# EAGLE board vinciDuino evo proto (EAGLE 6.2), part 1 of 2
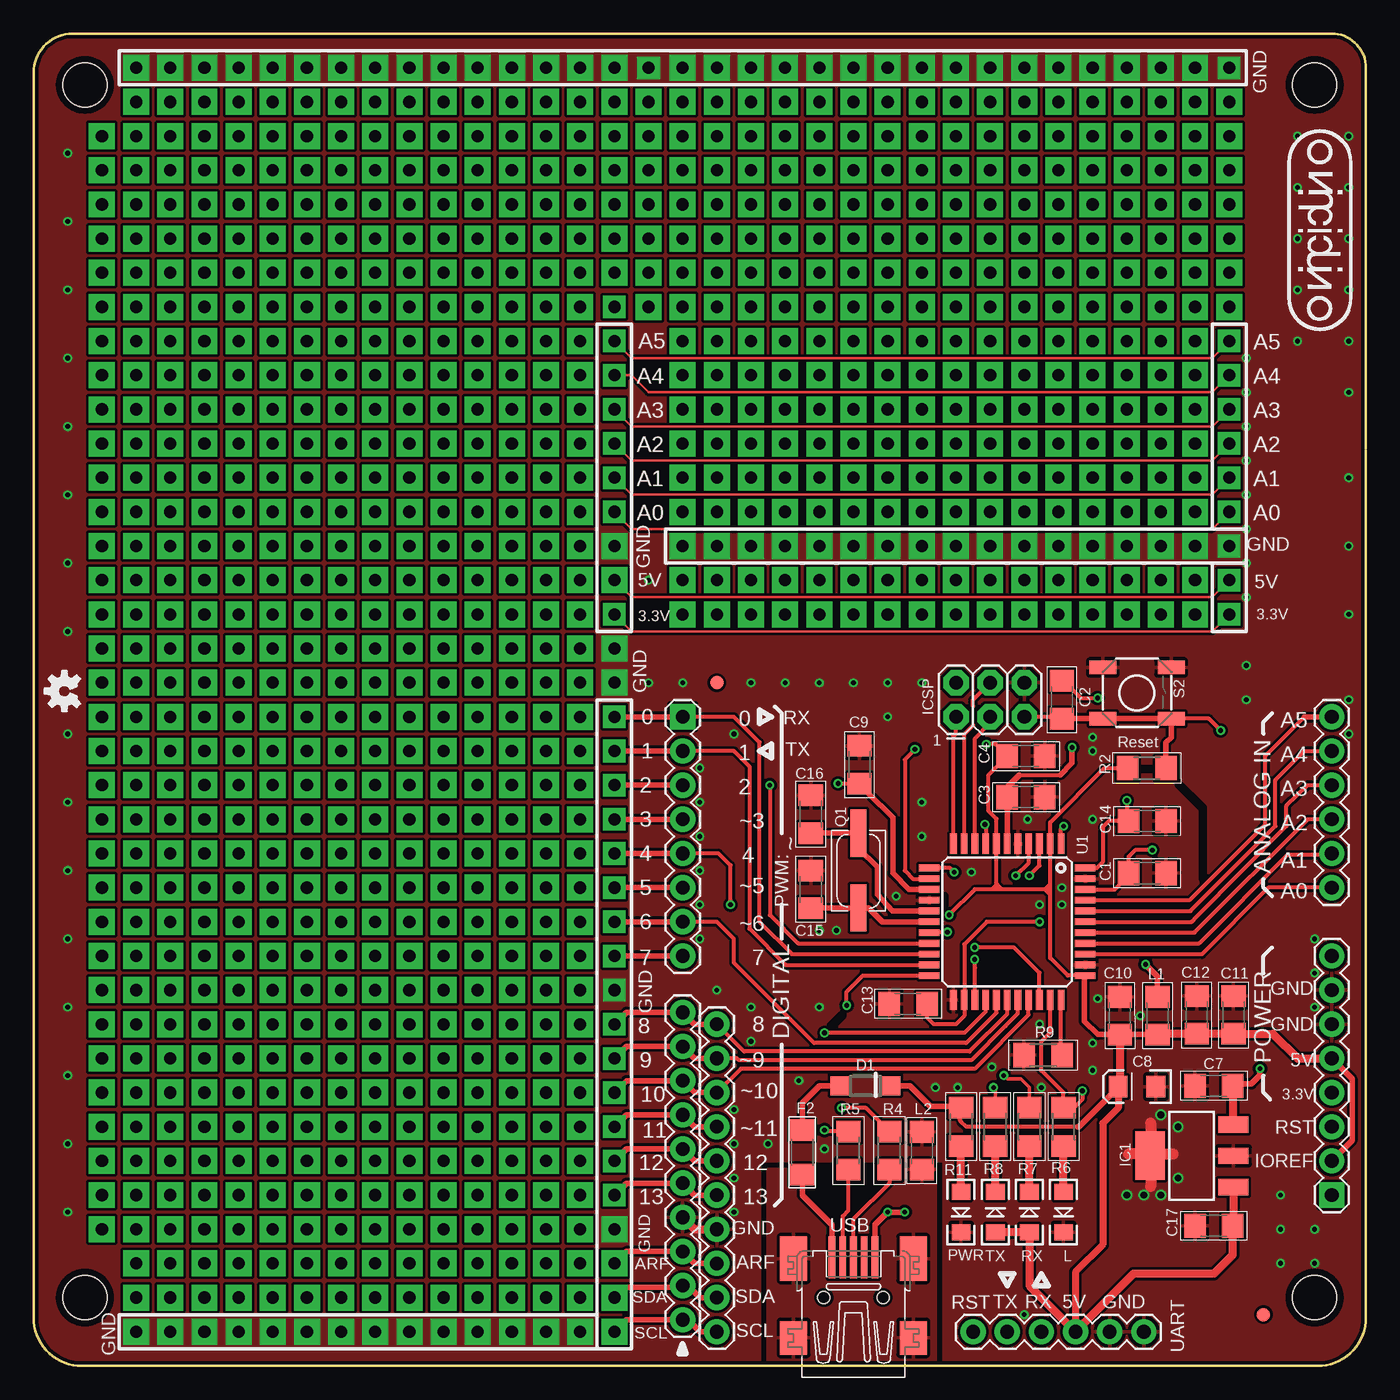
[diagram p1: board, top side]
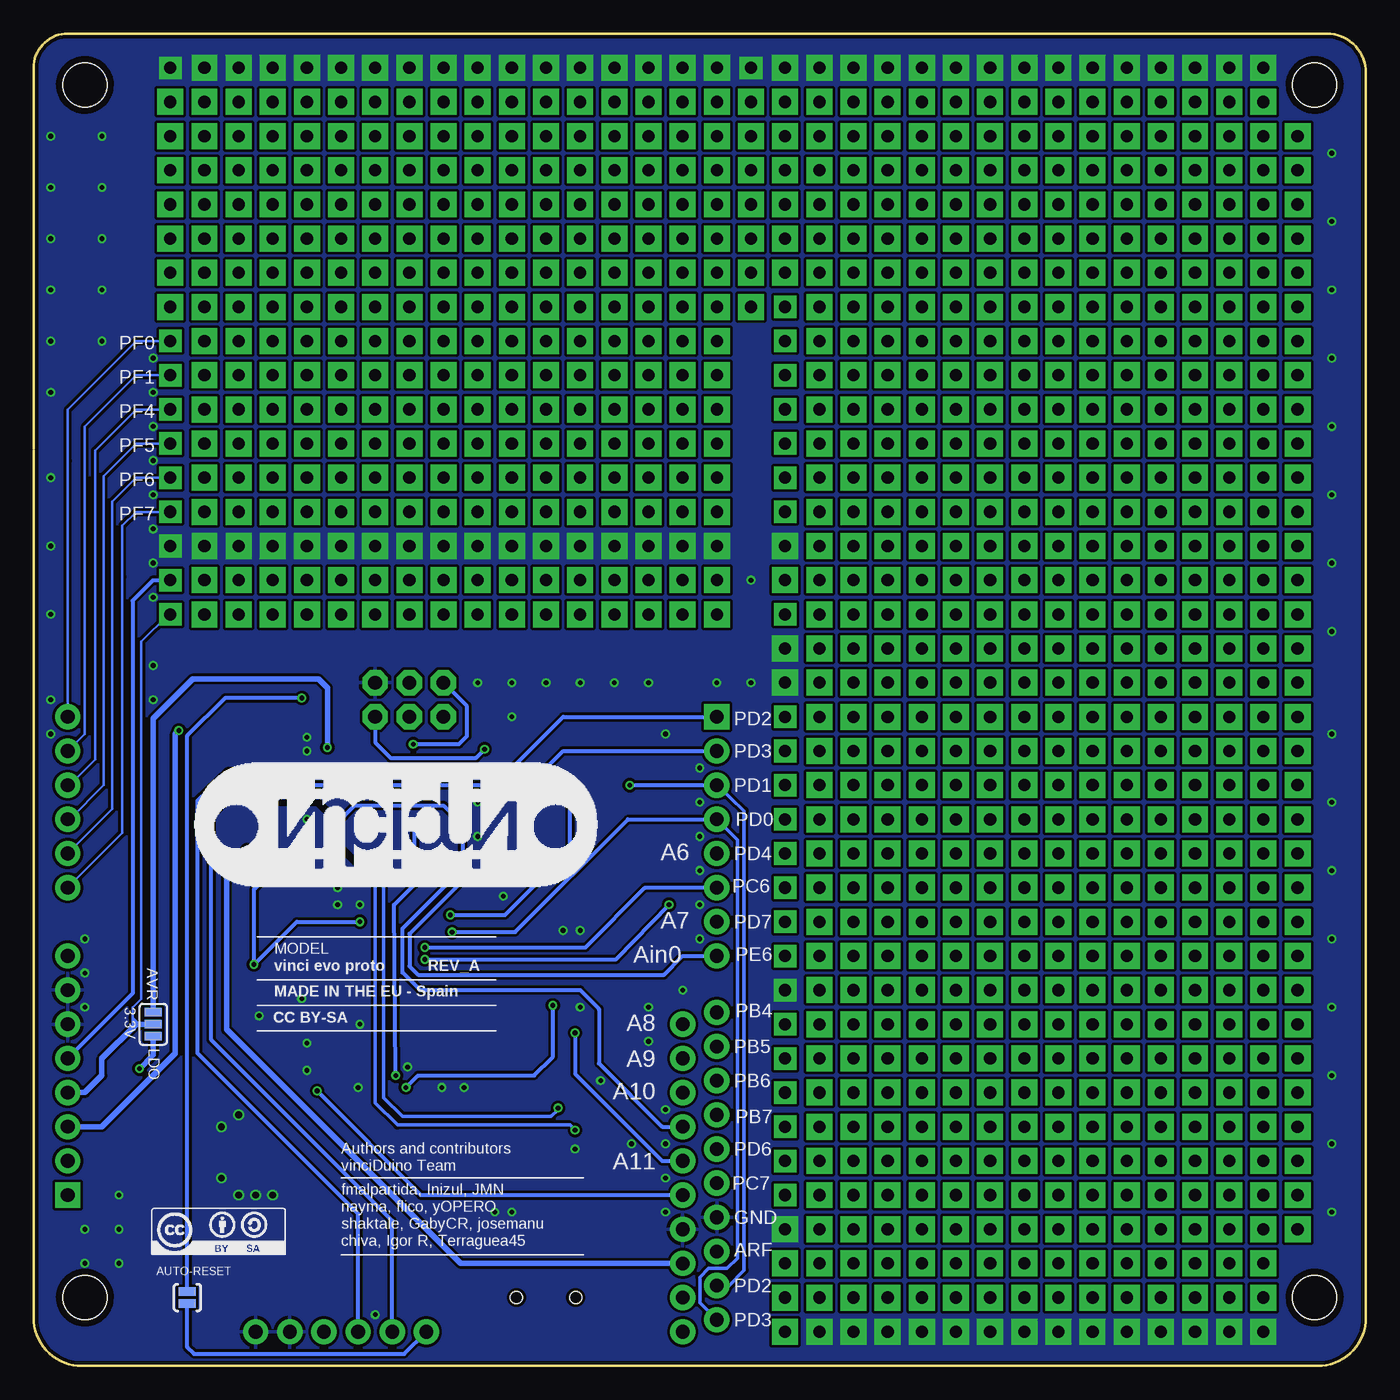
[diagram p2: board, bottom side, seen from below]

Size 99.06 x 99.06 mm. Coordinates in mm from the lower left corner, seen from the top.
Outline: 99.06,68.05 99.06,3.59 arc-90 95.47,0 3.59,0 arc-90 0,3.59 0,96.16 arc-90 2.9,99.06 96.52,99.06 arc-90 99.06,96.52 99.06,68.2
Copper layers (1*16): Top 0.0356mm / dielectric 1.5011mm / Bottom 0.0356mm
Design rules: minimum track width 6mil, minimum drill 0.35mm, track to track 8mil, track to pad 8mil, pad to pad 8mil, via to via 8mil, smd to smd 8mil, copper to edge 10mil, drill to drill 6mil, minimum pad ring 12mil, minimum via ring 6mil, stop-mask expansion 4mil, vias tented up to drill 25mil, thermal gap 10mil
Net classes: 1 vcc: width 0.254 mm; 2 usb: width 0.203 mm, clearance 0.508 mm
tRestrict: area 67.6,34.3 to 67.7,34.9; area 59.2,25.1 to 60.2,26.2; area 85.1,36.2 to 87,43.4; area 82.3,44.3 to 83.2,44.5
bRestrict: area 74.5,36.8 to 76.6,39.5; area 76.7,40.6 to 80.8,42

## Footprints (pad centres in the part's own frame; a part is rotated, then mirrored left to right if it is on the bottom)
SJ_3 = smd 0.635 x 1.27: 1 -0.889,0; 2 0,0; 3 0.889,0
SJ_2S-NO = smd 0.635 x 1.27: 1 -0.45,0; 2 0.45,0
1206 = smd 1.6 x 1.8: 1 -1.4,0; 2 1.4,0
EIA3216 = smd 1.4 x 1.6: A 1.4,0; C -1.4,0
SOD123 = smd 1.4 x 1.4: A 1.9,0; C -1.9,0
1206_PTC = smd 1.6 x 1.8: 1 -1.654,0; 2 1.654,0
SOT223 = smd 1.219 x 2.235: 1 -2.311,-3.099; 2 0,-3.099; 3 2.311,-3.099 | smd 3.6 x 2.2: 4 0,3.099
1X08@1 = drill 1.016 pad 1.88 square: 1 0,0 | drill 1.016 pad 1.88: 2 2.54,0; 3 5.08,0; 4 7.62,0; 5 10.16,0; 6 12.7,0; 7 15.24,0; 8 17.78,0
1X06@1 = drill 1.016 pad 1.88: 1 -6.35,0; 2 -3.81,0; 3 -1.27,0; 4 1.27,0; 5 3.81,0; 6 6.35,0
1X10 = drill 1.016 pad 1.88: 1 0,0; 2 2.54,0; 3 5.08,0; 4 7.62,0; 5 10.16,0; 6 12.7,0; 7 15.24,0; 8 17.78,0; 9 20.32,0; 10 22.86,0
2X3@1 = drill 1.016 pad 1.88 octagon: 1 0,0; 2 0,2.54; 3 2.54,0; 4 2.54,2.54; 5 5.08,0; 6 5.08,2.54
1X08 = drill 1.016 pad 1.88 square: 1 0,0 | drill 1.016 pad 1.88: 2 2.54,0; 3 5.08,0; 4 7.62,0; 5 10.16,0; 6 12.7,0; 7 15.24,0; 8 17.78,0
LED-1206 = smd 1.2 x 1.4: A -1.5,0; C 1.5,0
1206W = smd 1.6 x 1.8: 1 -1.4,0; 2 1.4,0
CSM-3X = smd 3.5 x 1.2: 1 2.775,0; 2 -2.775,0
R1206 = smd 1.6 x 1.803: 1 -1.422,0; 2 1.422,0
TACTILE_SWITCH_SMD@1 = smd 2 x 1: 1 -2.54,1.905; 2 2.54,1.905; 3 -2.54,-1.905; 4 2.54,-1.905
TQFP44 = smd 1.5 x 0.5: 1 -5.8,4; 2 -5.8,3.2; 3 -5.8,2.4; 4 -5.8,1.6; 5 -5.8,0.8; 6 -5.8,0; 7 -5.8,-0.8; 8 -5.8,-1.6; 9 -5.8,-2.4; 10 -5.8,-3.2; 11 -5.8,-4; 23 5.8,-4; 24 5.8,-3.2; 25 5.8,-2.4; 26 5.8,-1.6; 27 5.8,-0.8; 28 5.8,0; 29 5.8,0.8; 30 5.8,1.6; 31 5.8,2.4; 32 5.8,3.2; 33 5.8,4 | smd 0.5 x 1.5: 12 -4,-5.8; 13 -3.2,-5.8; 14 -2.4,-5.8; 15 -1.6,-5.8; 16 -0.8,-5.8; 17 0,-5.8; 18 0.8,-5.8; 19 1.6,-5.8; 20 2.4,-5.8; 21 3.2,-5.8; 22 4,-5.8; 34 4,5.8; 35 3.2,5.8; 36 2.4,5.8; 37 1.6,5.8; 38 0.8,5.8; 39 0,5.8; 40 -0.8,5.8; 41 -1.6,5.8; 42 -2.4,5.8; 43 -3.2,5.8; 44 -4,5.8
FIDUCIAL-1X2 = smd 1 x 1: 1 0,0
STAND-OFF@1 = hole 3.302: 0,0
32005-201 = smd 3.1 x 0.5: 1 3,1.6; 2 3,0.8; 3 3,0; 4 3,-0.8; 5 3,-1.6 | smd 2.5 x 2: M1 -3,-4.45; M2 -3,4.45 | smd 3.3 x 2: M3 2.9,4.45; M4 2.9,-4.45 | hole 0.9: 0,2.2; 0,-2.2

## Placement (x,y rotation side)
3.3V  [SJ_3]  90.17,25.4 270 bottom
AUTO-RESET  SOLDERJUMPERNO  [SJ_2S-NO]  87.63,5.08 90 bottom
C1  0.1uF  [1206]  82.8,36.64 180 top
C2  0.1uF  [1206]  76.45,49.53 270 top
C3  1uF  [1206]  73.79,42.29 0 top
C4  1uF  [1206]  73.79,45.34 0 top
C7  1uF  [1206]  87.76,20.83 180 top
C8  10uF  [EIA3216]  82.04,20.76 180 top
C9  0.1uF  [1206]  61.4,44.7 90 top
C10  0.1uF  [1206]  80.77,26.04 90 top
C11  10nF  [1206]  89.22,26.1 90 top
C12  1uF  [1206]  86.49,26.1 90 top
C13  0.1uF  [1206]  65.02,26.92 180 top
C14  0.1uF  [1206]  82.8,40.51 0 top
C15  18pF  [1206]  57.78,35.43 90 top
C16  18pF  [1206]  57.78,41.02 90 top
C17  0.1uF  [1206]  87.76,10.41 0 top
D1  MBR0520LT  [SOD123]  61.85,20.83 180 top
F2  1206L  [1206_PTC]  57.15,15.88 90 top
IC1  MCP1703  [SOT223]  86.11,15.62 90 top
J1  Digital  [1X08@1]  48.26,48.26 270 top
J2  Analog  [1X06@1]  96.52,41.91 90 top
JP1  Digital  [1X10]  48.26,26.29 270 top
JP2  Serial  [1X06@1]  76.2,2.54 0 top
JP3  ISP  [2X3@1]  68.59,48.26 0 top
JP4  [1X08]  96.52,12.7 90 top
JP5  Digital  [1X10]  50.8,25.4 270 top
L  Green  [LED-1206]  76.58,11.43 270 top
L1  Ferrite  [1206W]  83.57,26.04 90 top
L2  Ferrite  [1206W]  66.04,16 270 top
PWR  Red  [LED-1206]  68.96,11.43 270 top
Q1  CSM-3X-CRYSTALCSM-3X  [CSM-3X]  61.34,36.83 270 top
R2  10K  [R1206]  82.77,44.45 180 top
R4  22  [R1206]  63.63,16 270 top
R5  22  [R1206]  60.58,16 270 top
R6  1K  [R1206]  76.58,17.78 270 top
R7  1K  [R1206]  74.04,17.78 270 top
R8  1K  [R1206]  71.5,17.78 270 top
R9  10K  [R1206]  75.06,23.11 180 top
R11  2K2  [R1206]  68.96,17.78 90 top
REV_A  vinci evo proto  [ARDUINO_FORUM@1]  73.79,28.7 0 bottom
RX  Green  [LED-1206]  74.04,11.43 90 top
S2  Reset  [TACTILE_SWITCH_SMD@1]  82.04,50.04 0 top
TX  Green  [LED-1206]  71.5,11.43 90 top
U1  ATMEGA32U4-AU  [TQFP44]  72.39,33.02 270 top
U$1  VINCIDUINO_  [VINCIDUINO]  57.15,44.83 180 bottom
U$2  FIDUCIAL1X2  [FIDUCIAL-1X2]  91.44,3.81 90 top
U$3  VINCIDUINO_15  [VINCIDUINO_VSMAL]  98.04,76.96 90 top
U$4  FIDUCIAL1X2  [FIDUCIAL-1X2]  50.8,50.8 90 top
U$5  STAND-OFF  [STAND-OFF@1]  95.25,5.08 90 top
U$9  STAND-OFF  [STAND-OFF@1]  3.81,95.25 90 top
U$10  STAND-OFF  [STAND-OFF@1]  95.25,95.25 90 top
U$13  [SA-BY]  90.3,8.26 0 bottom
U$14  OSHW-LOGOS  [OSHW-LOGO-S]  2.29,50.16 90 top
U$15  STAND-OFF  [STAND-OFF@1]  3.81,5.08 90 top
USB  MINI-USB-SCHIELD-32005-201  [32005-201]  60.96,5.08 90 top

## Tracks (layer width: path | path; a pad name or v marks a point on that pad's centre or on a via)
3.3V  (via drill 0.9 pad 1.68)
  Top 0.203: v43.18,55.88 44.45,54.61 87.63,54.61 v88.9,55.88
  Bottom 0.203: v88.9,55.88 89.03,55.88 91.06,53.85 91.06,27.3 91.69,26.67 91.69,25.91 | 91.69,25.91 91.19,25.4 | 91.69,25.91 91.69,25.27 91.57,25.27 91.57,25.65
  Bottom 0.406: JP4.4 95.25,20.32 93.98,21.59 93.98,22.86 91.44,25.4 91.19,25.4 3.3V.2
A0  (via drill 0.9 pad 1.68)
  Top 0.203: v43.18,63.5 44.45,62.23 87.63,62.23 v88.9,63.5
  Top 0.305: J2.1 91.82,35.56 86.87,30.61 86.86,30.62 U1.36
  Bottom 0.203: J2.1 92.46,39.62 92.46,58.67 92.46,62.48 91.44,63.5 v88.9,63.5
A1  (via drill 0.9 pad 1.68)
  Top 0.203: v43.18,66.04 44.45,64.77 87.63,64.77 v88.9,66.04
  Top 0.305: J2.2 96.39,37.97 93.22,37.97 86.67,31.42 U1.37
  Bottom 0.203: J2.2 93.22,41.4 93.22,60.45 93.22,64.26 91.44,66.04 v88.9,66.04
A2  (via drill 0.9 pad 1.68)
  Top 0.203: v43.18,68.58 44.45,67.31 87.63,67.31 v88.9,68.58
  Top 0.305: J2.3 94.74,40.64 86.32,32.22 U1.38
  Bottom 0.203: J2.3 96.39,40.64 93.85,43.18 93.85,62.36 93.85,66.17 91.44,68.58 v88.9,68.58
A3  (via drill 0.9 pad 1.68)
  Top 0.203: v43.18,71.12 44.45,69.85 87.63,69.85 v88.9,71.12
  Top 0.305: J2.4 94.74,43.18 93.15,41.66 93.15,40.13 86.49,33.4 86.11,33.02 U1.39
  Bottom 0.203: J2.4 96.39,43.18 94.49,45.09 94.49,64.26 94.49,68.07 91.44,71.12 v88.9,71.12
A4  (via drill 0.9 pad 1.68)
  Top 0.203: v43.18,73.66 44.45,73.66 45.72,72.39 87.63,72.39 v88.9,73.66
  Top 0.305: 78.23,33.78 U1.40 86.02,33.82 92.33,40.13 92.33,43.56 94.49,45.72 J2.5
  Bottom 0.203: J2.5 95.25,46.99 95.25,66.04 95.25,69.85 91.44,73.66 v88.9,73.66
A5  (via drill 0.9 pad 1.68)
  Top 0.203: v43.18,76.2 44.45,74.93 87.63,74.93 v88.9,76.2
  Top 0.305: U1.41 85.93,34.62 91.57,40.26 91.57,45.34 94.49,48.26
  Top 0.406: 94.49,48.26 J2.6
  Bottom 0.203: J2.6 96.52,67.31 96.52,71.12 91.44,76.2 v88.9,76.2
AREF  (via drill 0.35, 0.9 pad 1.93)
  Top 0.305: U1.42 80.38,35.42 81.53,36.58 81.53,36.64 C1.2 81.41,37.85 81.92,38.35 v83.19,38.35
  Top 0.406: JP5.8 49.15,7.62 JP1.8 44.07,8.51 v43.18,7.62
  Bottom 0.406: v83.19,38.35 84.71,36.83 84.71,25.02 67.31,7.62 JP5.8
AVCC  (via drill 0.35)
  Top 0.305: U1.44 79.06,37.02 79.5,37.47 79.5,40.07 79.95,40.51 C14.1 81.28,40.51 v81.28,42.04 | C13.1 66.42,25.91 66.93,25.4 68.58,25.4 69.19,26.01 U1.24 69.19,31.34 70.87,33.02 v74.8,33.02
  Top 0.406: v82.68,29.84 83.57,28.96 L1.2
  Bottom 0.305: v74.8,33.02 79.5,33.02 v82.68,29.84 82.68,35.43 81.28,36.83 v81.28,42.04
D2/SDA  (via drill 0.35, 0.9 pad 1.68, 0.9 pad 1.93)
  Top 0.305: U1.19 56.84,31.42 54.74,33.53 v54.74,43.18
  Top 0.406: JP5.9 49.53,5.08 48.64,5.97 JP1.9 48.13,5.84 44.07,5.84 43.31,5.08 v43.18,5.08 | J1.3 v43.18,43.18
  Bottom 0.254: JP1.9 47.37,5.97 46.23,7.11 46.23,41.27 J1.3
  Bottom 0.305: v54.74,43.18 J1.3
D3/SCL  (via drill 0.35, 0.9 pad 1.68, 0.9 pad 1.93)
  Top 0.305: U1.18 68.03,32.22 v67.94,32.26
  Top 0.406: JP5.10 49.53,2.54 48.64,3.43 JP1.10 44.07,3.43 v43.18,2.54 | J1.4 v43.18,40.64
  Bottom 0.254: J1.4 46.74,39.12 46.74,8 47.5,7.24 48.9,7.24 49.53,6.6 49.53,4.7 JP1.10
  Bottom 0.305: v67.94,32.26 63.25,32.26 54.86,40.64 J1.4
D4  (via drill 0.35, 0.9 pad 1.68)
  Top 0.305: U1.25 69.99,29.6 v69.98,30.23 | v51.82,34.29 51.82,37.21 50.93,38.1 J1.5
  Top 0.406: J1.5 v43.18,38.1
  Bottom 0.305: v69.98,30.23 55.75,30.23 v51.82,34.29
D5  (via drill 0.35, 0.9 pad 1.68)
  Top 0.305: U1.31 74.79,29.22 72.9,31.11 v69.98,31.11
  Top 0.406: J1.6 v43.18,35.56
  Bottom 0.305: v69.98,31.11 58.04,31.11 53.59,35.56 J1.6
D6  (via drill 0.9 pad 1.68)
  Top 0.305: 71.59,26.5 U1.27 71.59,26.25 69.34,24 58.04,24 52.07,29.97 52.07,31.75 50.8,33.02 J1.7
  Top 0.406: J1.7 v43.18,33.02
D7  (via drill 0.35, 0.9 pad 1.68)
  Top 0.305: U1.1 76.39,39.94 v76.58,40.13
  Top 0.406: J1.8 v43.18,30.48
  Bottom 0.305: v76.58,40.13 76.58,40.26 75.18,41.66 68.58,41.66 67.18,40.26 67.18,36.07 71.12,32.13 71.12,29.72 70.48,29.08 52.2,29.08 50.8,30.48 J1.8
D8  (via drill 0.9 pad 1.68)
  Top 0.305: U1.28 72.39,26.16 69.6,23.37 52.83,23.37 JP5.1
  Top 0.406: JP5.1 49.15,25.4 JP1.1 44.07,26.29 v43.18,25.4
D9  (via drill 0.9 pad 1.68)
  Top 0.305: 72.26,25.27 69.72,22.73 52.45,22.73 52.32,22.86 JP5.2 | 72.26,25.27 | 72.26,25.27 73.18,26.19 U1.29
  Top 0.406: JP5.2 49.15,22.86 JP1.2 44.07,23.75 v43.18,22.86
D10  (via drill 0.9 pad 1.68)
  Top 0.305: U1.30 73.98,27.21 73.98,26.1 69.98,22.1 52.58,22.1 JP5.3
  Top 0.406: JP5.3 49.15,20.32 JP1.3 44.07,21.21 v43.18,20.32
D11  (via drill 0.35, 0.9 pad 1.68)
  Top 0.305: U1.12 68.14,37.02 v68.45,36.7
  Top 0.406: JP5.4 49.15,17.78 JP1.4 44.07,18.67 v43.18,17.78
  Bottom 0.305: v68.45,36.7 68.45,35.69 71.63,32.51 71.63,29.24 70.33,27.94 58.42,27.94 57.02,26.54 57.02,22.48 52.32,17.78 JP5.4
D12  (via drill 0.35, 0.9 pad 1.68)
  Top 0.305: U1.26 70.79,26.34 69.22,24.77 v58.8,24.77
  Top 0.406: JP5.5 49.15,15.24 JP1.5 44.07,16.13 v43.18,15.24
  Bottom 0.305: v58.8,24.77 58.8,21.72 52.32,15.24 JP5.5
D13  (via drill 0.35, 0.9 pad 1.68)
  Top 0.305: U1.32 75.59,24.79 74.93,24.13 74.93,21.97 76.58,20.32 R6.1 76.22,19.18 77.34,19.18 77.98,19.81 v77.98,20.45
  Top 0.406: JP5.6 49.15,12.7 JP1.6 44.07,13.59 v43.18,12.7
  Bottom 0.305: v77.98,20.45 70.23,12.7 JP5.6
D+  (via drill 0.35)
  Top 0.305: U1.4 73.99,37.41 v73.03,36.45 | 63.6,17.42 R4.1 61.87,19.18 v60.07,19.18
  Bottom 0.254: 60.07,19.05 60.58,18.54 71.63,18.54 73.03,19.94 v73.03,36.45
  Bottom 0.305: v60.07,19.18 60.07,19.05
D-  (via drill 0.35)
  Top 0.305: U1.3 74.79,37.2 v74.04,36.45 | R5.1 58.9,17.42 v58.8,17.53
  Bottom 0.254: v74.04,36.45 73.66,36.07 73.66,19.56 72.01,17.91 59.18,17.91 v58.8,17.53
GND  (via drill 0.35, 0.5, 0.9 pad 1.68, 0.9 pad 1.93)
  Top 0.406: USB.5 62.56,10.49 v63.5,11.43 v64.77,11.43
  Top 0.61: 48.39,10.92 49.15,10.16 JP5.7
  Top 0.813: 83.06,18.03 83.06,17.14 | 83.82,15.75 84.71,15.75 | 83.06,14.35 83.06,13.34 | 82.04,15.75 81.41,15.75
  other vias: 71.25,22.23 78.74,24 78.74,21.97 53.34,24.13 49.53,39.37 53.34,26.67 2.54,69.85 52.07,11.43 49.53,34.29 52.07,46.99 66.04,39.37 66.04,41.91 49.53,41.91 52.07,13.97 54.61,16.51 95.25,26.67 95.25,29.21 58.42,26.67 78.74,45.72 78.74,46.74 73.91,40.64 74.8,34.29 69.72,36.7 76.45,34.29 76.45,35.56 79.12,27.3 82.3,26.04 78.74,40.64 68.71,20.7 49.53,44.45 49.53,36.83 49.53,31.75 52.07,16.51 52.07,19.05 95.25,31.75 74.8,25.4 74.93,20.7 59.69,32.38 64.14,34.92 58.42,32.38 92.71,10.16 92.71,12.7 88.9,60.96 83.82,60.96 81.28,60.96 78.74,60.96 76.2,60.96 73.66,60.96 71.12,60.96 68.58,60.96 66.04,60.96 63.5,60.96 60.96,60.96 58.42,60.96 55.88,60.96 53.34,60.96 50.8,60.96 48.26,60.96 43.18,27.94 43.18,10.16 92.71,7.62 95.25,10.16 95.25,7.62 85.09,17.78 85.09,13.97 45.72,58.42 53.34,50.8 55.88,50.8 58.42,50.8 60.96,50.8 63.5,50.8 66.04,50.8 63.5,48.26 93.98,76.2 90.17,74.93 90.17,72.39 90.17,69.85 90.17,67.31 90.17,64.77 90.17,62.23 90.17,59.69 90.17,57.15 97.79,66.04 97.79,60.96 97.79,55.88 97.79,46.99 97.79,49.53 2.54,64.77 2.54,54.61 2.54,46.99 2.54,41.91 2.54,36.83 2.54,31.75 2.54,26.67 2.54,21.59 2.54,16.51 2.54,11.43 45.72,50.8 48.26,50.8 73.66,3.81 56.9,21.21 67.06,20.7 50.8,27.94 90.17,52.07 90.17,49.53 43.18,60.96 43.18,53.34 43.18,50.8 45.72,96.52 43.18,96.52 40.64,96.52 38.1,96.52 35.56,96.52 33.02,96.52 30.48,96.52 27.94,96.52 25.4,96.52 22.86,96.52 20.32,96.52 17.78,96.52 15.24,96.52 12.7,96.52 10.16,96.52 7.62,96.52 88.9,96.52 83.82,96.52 81.28,96.52 78.74,96.52 76.2,96.52 73.66,96.52 71.12,96.52 68.58,96.52 66.04,96.52 63.5,96.52 60.96,96.52 58.42,96.52 55.88,96.52 53.34,96.52 50.8,96.52 48.26,96.52 40.64,2.54 38.1,2.54 35.56,2.54 33.02,2.54 30.48,2.54 27.94,2.54 25.4,2.54 22.86,2.54 20.32,2.54 17.78,2.54 15.24,2.54 12.7,2.54 10.16,2.54 7.62,2.54 58.8,16.13 86.36,60.96 86.36,96.52 97.79,72.39 97.79,76.2 2.54,59.69 2.54,74.93 2.54,80.01 2.54,85.09 2.54,90.17 93.98,80.01 97.79,80.01 97.79,83.82 93.98,83.82 93.98,87.63 97.79,87.63 97.79,91.44 93.98,91.44 83.82,12.7 82.55,12.7 81.28,12.7 83.82,18.67
  pour Top (isolate 0.203): 0,0 0,99.06 99.06,99.06 99.06,0 67.69,0.25 67.69,15.24 53.98,15.24 53.98,0
  pour Bottom (isolate 0.203): 0,0 0,99.06 99.06,99.06 98.93,15.88 98.93,10.79 99.06,0
MISO
  Top 0.305: U1.11 68.39,46.8 68.58,46.99 JP3.1
MOSI
  Top 0.203: 69.85,47.62 69.85,49.05
  Top 0.305: U1.10 69.22,38.84 69.22,46.99 69.72,47.5 69.85,47.62 | 69.85,49.05 69.85,49.52 JP3.4
N$1
  Top 0.61: TX.C R8.2
N$2
  Top 0.305: USB.2 60.16,11.14 60.58,11.56 R5.2
N$3
  Top 0.406: C16.1 61.33,39.62 Q1.2 61.34,38.48 62.74,37.08 62.74,35.05 63.84,33.82 U1.16
N$4
  Top 0.406: C15.1 61.34,34.03 61.34,34.04 Q1.1 62.08,34.05 63.12,33.02 U1.17
N$5
  Top 0.305: R4.2 63.63,13.59 60.96,10.92 USB.3
N$6
  Top 0.305: U1.33 76.39,23.2 R9.1
N$7
  Top 0.61: L.A R6.2
N$8  (via drill 0.35)
  Top 0.305: C2.1 76.58,50.93 77.85,49.66 v79.12,49.66
  Bottom 0.305: AUTO-RESET.2 87.63,46.86 84.84,49.66 v79.12,49.66
N$9
  Top 0.61: RX.C R7.2
N$10
  pour Top: 54.61,14.61 67.06,14.61 67.06,0 54.61,0
N$12  (via drill 0.9 pad 1.93)
  other vias: 83.82,76.2
N$13
  Top 0.406: USB.1 59.36,10.49 57.15,12.7 F2.1
N$14  (via drill 0.9 pad 1.93)
  other vias: 83.82,73.66
N$16  (via drill 0.9 pad 1.93)
  other vias: 83.82,71.12
N$17  (via drill 0.9 pad 1.93)
  other vias: 83.82,68.58
N$18  (via drill 0.9 pad 1.93)
  other vias: 83.82,66.04
N$21  (via drill 0.9 pad 1.93)
  other vias: 83.82,63.5
N$36
  Top 0.406: F2.2 57.15,19.56 58.42,20.83 D1.A
N$37  (via drill 0.9 pad 1.93)
  other vias: 83.82,58.42
N$38
  Top 0.61: PWR.A R11.1
N$48  (via drill 0.9 pad 1.93)
  other vias: 83.82,55.88
N$49  (via drill 0.9 pad 1.93)
  other vias: 81.28,55.88
N$50  (via drill 0.9 pad 1.93)
  other vias: 81.28,58.42
N$52  (via drill 0.9 pad 1.93)
  other vias: 38.1,53.34
N$53  (via drill 0.9 pad 1.93)
  other vias: 81.28,63.5
N$54  (via drill 0.9 pad 1.93)
  other vias: 81.28,66.04
N$55  (via drill 0.9 pad 1.93)
  other vias: 81.28,68.58
N$56  (via drill 0.9 pad 1.93)
  other vias: 81.28,71.12
N$58  (via drill 0.9 pad 1.93)
  other vias: 81.28,73.66
N$59  (via drill 0.9 pad 1.93)
  other vias: 81.28,76.2
N$60  (via drill 0.9 pad 1.93)
  other vias: 78.74,76.2
N$62  (via drill 0.9 pad 1.93)
  other vias: 78.74,73.66
N$63  (via drill 0.9 pad 1.93)
  other vias: 78.74,71.12
N$65  (via drill 0.9 pad 1.93)
  other vias: 78.74,68.58
N$66  (via drill 0.9 pad 1.93)
  other vias: 78.74,66.04
N$67  (via drill 0.9 pad 1.93)
  other vias: 78.74,63.5
N$70  (via drill 0.9 pad 1.93)
  other vias: 35.56,53.34
N$71  (via drill 0.9 pad 1.93)
  other vias: 78.74,58.42
N$72  (via drill 0.9 pad 1.93)
  other vias: 78.74,55.88
N$75  (via drill 0.9 pad 1.93)
  other vias: 76.2,55.88
N$76  (via drill 0.9 pad 1.93)
  other vias: 76.2,58.42
N$77  (via drill 0.9 pad 1.93)
  other vias: 33.02,53.34
N$82  (via drill 0.9 pad 1.93)
  other vias: 76.2,63.5
N$87  (via drill 0.9 pad 1.93)
  other vias: 76.2,66.04
N$88  (via drill 0.9 pad 1.93)
  other vias: 76.2,68.58
N$90  (via drill 0.9 pad 1.93)
  other vias: 76.2,71.12
N$92  (via drill 0.9 pad 1.93)
  other vias: 76.2,73.66
N$93  (via drill 0.9 pad 1.93)
  other vias: 76.2,76.2
N$94  (via drill 0.35)
  Top 0.305: 73.28,43.94 76.33,43.94 | 72.39,41.91 C3.1
  Top 0.406: U1.6 72.39,41.91 72.39,43.05 73.28,43.94 | 76.33,43.94 77.22,44.83 v77.22,45.97
  Bottom 0.406: v77.22,45.97 77.22,50.42 77.85,51.05 87.25,51.05 90.17,48.13 3.3V.1
N$99  (via drill 0.9 pad 1.93)
  other vias: 73.66,76.2
N$103  (via drill 0.9 pad 1.93)
  other vias: 73.66,73.66
N$107  (via drill 0.9 pad 1.93)
  other vias: 73.66,71.12
N$108  (via drill 0.9 pad 1.93)
  other vias: 73.66,68.58
N$109  (via drill 0.9 pad 1.93)
  other vias: 73.66,66.04
N$110  (via drill 0.9 pad 1.93)
  other vias: 73.66,63.5
N$111  (via drill 0.9 pad 1.93)
  other vias: 30.48,53.34
N$116  (via drill 0.9 pad 1.93)
  other vias: 73.66,58.42
N$121  (via drill 0.9 pad 1.93)
  other vias: 73.66,55.88
N$122  (via drill 0.9 pad 1.93)
  other vias: 71.12,55.88
N$124  (via drill 0.9 pad 1.93)
  other vias: 71.12,58.42
N$125  (via drill 0.9 pad 1.93)
  other vias: 27.94,53.34
N$126  (via drill 0.9 pad 1.93)
  other vias: 71.12,63.5
N$127  (via drill 0.9 pad 1.93)
  other vias: 71.12,66.04
N$128  (via drill 0.9 pad 1.93)
  other vias: 71.12,68.58
N$132  (via drill 0.9 pad 1.93)
  other vias: 71.12,71.12
N$133  (via drill 0.9 pad 1.93)
  other vias: 71.12,73.66
N$136  (via drill 0.9 pad 1.93)
  other vias: 71.12,76.2
N$138  (via drill 0.9 pad 1.93)
  other vias: 25.4,53.34
N$139  (via drill 0.9 pad 1.93)
  other vias: 22.86,53.34
N$140  (via drill 0.9 pad 1.93)
  other vias: 20.32,53.34
N$141  (via drill 0.9 pad 1.93)
  other vias: 17.78,53.34
N$142  (via drill 0.9 pad 1.93)
  other vias: 15.24,53.34
N$143  (via drill 0.9 pad 1.93)
  other vias: 12.7,53.34
N$144  (via drill 0.9 pad 1.93)
  other vias: 10.16,53.34
N$145  (via drill 0.9 pad 1.93)
  other vias: 7.62,53.34
N$148  (via drill 0.9 pad 1.93)
  other vias: 5.08,53.34
N$150  (via drill 0.9 pad 1.93)
  other vias: 40.64,58.42
N$152  (via drill 0.9 pad 1.93)
  other vias: 40.64,30.48
N$154  (via drill 0.9 pad 1.93)
  other vias: 40.64,33.02
N$155  (via drill 0.9 pad 1.93)
  other vias: 40.64,35.56
N$157  (via drill 0.9 pad 1.93)
  other vias: 40.64,38.1
N$158  (via drill 0.9 pad 1.93)
  other vias: 40.64,40.64
N$159  (via drill 0.9 pad 1.93)
  other vias: 40.64,43.18
N$160  (via drill 0.9 pad 1.93)
  other vias: 40.64,45.72
N$161  (via drill 0.9 pad 1.93)
  other vias: 40.64,48.26
N$162  (via drill 0.9 pad 1.93)
  other vias: 38.1,48.26
N$163  (via drill 0.9 pad 1.93)
  other vias: 38.1,45.72
N$167  (via drill 0.9 pad 1.93)
  other vias: 38.1,43.18
N$169  (via drill 0.9 pad 1.93)
  other vias: 38.1,40.64
N$172  (via drill 0.9 pad 1.93)
  other vias: 38.1,38.1
N$174  (via drill 0.9 pad 1.93)
  other vias: 38.1,35.56
N$176  (via drill 0.9 pad 1.93)
  other vias: 38.1,33.02
N$177  (via drill 0.9 pad 1.93)
  other vias: 38.1,30.48
N$178  (via drill 0.9 pad 1.93)
  other vias: 40.64,78.74
N$179  (via drill 0.9 pad 1.93)
  other vias: 38.1,50.8
N$183  (via drill 0.9 pad 1.93)
  other vias: 35.56,30.48
N$184  (via drill 0.9 pad 1.93)
  other vias: 35.56,33.02
N$186  (via drill 0.9 pad 1.93)
  other vias: 35.56,35.56
N$190  (via drill 0.9 pad 1.93)
  other vias: 35.56,38.1
N$193  (via drill 0.9 pad 1.93)
  other vias: 35.56,40.64
N$194  (via drill 0.9 pad 1.93)
  other vias: 35.56,43.18
N$195  (via drill 0.9 pad 1.93)
  other vias: 35.56,45.72
N$196  (via drill 0.9 pad 1.93)
  other vias: 35.56,48.26
N$200  (via drill 0.9 pad 1.93)
  other vias: 33.02,48.26
N$201  (via drill 0.9 pad 1.93)
  other vias: 33.02,45.72
N$203  (via drill 0.9 pad 1.93)
  other vias: 33.02,43.18
N$208  (via drill 0.9 pad 1.93)
  other vias: 33.02,40.64
N$210  (via drill 0.9 pad 1.93)
  other vias: 33.02,38.1
N$211  (via drill 0.9 pad 1.93)
  other vias: 33.02,35.56
N$212  (via drill 0.9 pad 1.93)
  other vias: 33.02,33.02
N$213  (via drill 0.9 pad 1.93)
  other vias: 33.02,30.48
N$214  (via drill 0.9 pad 1.93)
  other vias: 35.56,50.8
N$217  (via drill 0.9 pad 1.93)
  other vias: 33.02,50.8
N$218  (via drill 0.9 pad 1.93)
  other vias: 30.48,30.48
N$219  (via drill 0.9 pad 1.93)
  other vias: 30.48,33.02
N$220  (via drill 0.9 pad 1.93)
  other vias: 30.48,35.56
N$222  (via drill 0.9 pad 1.93)
  other vias: 30.48,38.1
N$225  (via drill 0.9 pad 1.93)
  other vias: 30.48,40.64
N$226  (via drill 0.9 pad 1.93)
  other vias: 30.48,43.18
N$228  (via drill 0.9 pad 1.93)
  other vias: 30.48,45.72
N$229  (via drill 0.9 pad 1.93)
  other vias: 30.48,48.26
N$230  (via drill 0.9 pad 1.93)
  other vias: 30.48,50.8
N$231  (via drill 0.9 pad 1.93)
  other vias: 27.94,50.8
N$232  (via drill 0.9 pad 1.93)
  other vias: 25.4,50.8
N$233  (via drill 0.9 pad 1.93)
  other vias: 22.86,50.8
N$235  (via drill 0.9 pad 1.93)
  other vias: 20.32,50.8
N$240  (via drill 0.9 pad 1.93)
  other vias: 17.78,50.8
N$241  (via drill 0.9 pad 1.93)
  other vias: 15.24,50.8
N$243  (via drill 0.9 pad 1.93)
  other vias: 12.7,50.8
N$244  (via drill 0.9 pad 1.93)
  other vias: 10.16,50.8
N$245  (via drill 0.9 pad 1.93)
  other vias: 40.64,5.08
N$246  (via drill 0.9 pad 1.93)
  other vias: 40.64,7.62
N$247  (via drill 0.9 pad 1.93)
  other vias: 40.64,10.16
N$251  (via drill 0.9 pad 1.93)
  other vias: 40.64,12.7
N$252  (via drill 0.9 pad 1.93)
  other vias: 40.64,15.24
N$257  (via drill 0.9 pad 1.93)
  other vias: 40.64,17.78
N$258  (via drill 0.9 pad 1.93)
  other vias: 40.64,20.32
N$259  (via drill 0.9 pad 1.93)
  other vias: 40.64,22.86
N$266  (via drill 0.9 pad 1.93)
  other vias: 40.64,25.4
N$267  (via drill 0.9 pad 1.93)
  other vias: 38.1,25.4
N$269  (via drill 0.9 pad 1.93)
  other vias: 38.1,22.86
N$270  (via drill 0.9 pad 1.93)
  other vias: 38.1,20.32
N$277  (via drill 0.9 pad 1.93)
  other vias: 38.1,17.78
N$279  (via drill 0.9 pad 1.93)
  other vias: 38.1,15.24
N$280  (via drill 0.9 pad 1.93)
  other vias: 38.1,12.7
N$281  (via drill 0.9 pad 1.93)
  other vias: 38.1,10.16
N$282  (via drill 0.9 pad 1.93)
  other vias: 38.1,7.62
N$283  (via drill 0.9 pad 1.93)
  other vias: 38.1,5.08
N$284  (via drill 0.9 pad 1.93)
  other vias: 35.56,5.08
N$286  (via drill 0.9 pad 1.93)
  other vias: 35.56,7.62
N$289  (via drill 0.9 pad 1.93)
  other vias: 35.56,10.16
N$292  (via drill 0.9 pad 1.93)
  other vias: 35.56,12.7
N$293  (via drill 0.9 pad 1.93)
  other vias: 35.56,15.24
N$294  (via drill 0.9 pad 1.93)
  other vias: 35.56,17.78
N$295  (via drill 0.9 pad 1.93)
  other vias: 35.56,20.32
N$296  (via drill 0.9 pad 1.93)
  other vias: 35.56,22.86
N$297  (via drill 0.9 pad 1.93)
  other vias: 35.56,25.4
N$298  (via drill 0.9 pad 1.93)
  other vias: 33.02,25.4
N$299  (via drill 0.9 pad 1.93)
  other vias: 33.02,22.86
N$300  (via drill 0.9 pad 1.93)
  other vias: 33.02,20.32
N$301  (via drill 0.9 pad 1.93)
  other vias: 33.02,17.78
N$302  (via drill 0.9 pad 1.93)
  other vias: 33.02,15.24
N$303  (via drill 0.9 pad 1.93)
  other vias: 33.02,12.7
N$304  (via drill 0.9 pad 1.93)
  other vias: 33.02,10.16
N$305  (via drill 0.9 pad 1.93)
  other vias: 33.02,7.62
N$306  (via drill 0.9 pad 1.93)
  other vias: 33.02,5.08
N$307  (via drill 0.9 pad 1.93)
  other vias: 30.48,5.08
N$308  (via drill 0.9 pad 1.93)
  other vias: 30.48,7.62
N$309  (via drill 0.9 pad 1.93)
  other vias: 30.48,10.16
N$310  (via drill 0.9 pad 1.93)
  other vias: 30.48,12.7
N$311  (via drill 0.9 pad 1.93)
  other vias: 30.48,15.24
N$312  (via drill 0.9 pad 1.93)
  other vias: 30.48,17.78
N$313  (via drill 0.9 pad 1.93)
  other vias: 30.48,20.32
N$314  (via drill 0.9 pad 1.93)
  other vias: 30.48,22.86
N$315  (via drill 0.9 pad 1.93)
  other vias: 30.48,25.4
N$316  (via drill 0.9 pad 1.93)
  other vias: 68.58,76.2
N$317  (via drill 0.9 pad 1.93)
  other vias: 68.58,73.66
N$318  (via drill 0.9 pad 1.93)
  other vias: 68.58,71.12
N$319  (via drill 0.9 pad 1.93)
  other vias: 68.58,68.58
N$320  (via drill 0.9 pad 1.93)
  other vias: 68.58,66.04
N$321  (via drill 0.9 pad 1.93)
  other vias: 68.58,63.5
N$322  (via drill 0.9 pad 1.93)
  other vias: 7.62,50.8
N$323  (via drill 0.9 pad 1.93)
  other vias: 68.58,58.42
N$324  (via drill 0.9 pad 1.93)
  other vias: 68.58,55.88
N$327  (via drill 0.9 pad 1.93)
  other vias: 66.04,55.88
N$329  (via drill 0.9 pad 1.93)
  other vias: 66.04,58.42
N$331  (via drill 0.9 pad 1.93)
  other vias: 5.08,50.8
N$332  (via drill 0.9 pad 1.93)
  other vias: 66.04,63.5
N$333  (via drill 0.9 pad 1.93)
  other vias: 66.04,66.04
N$334  (via drill 0.9 pad 1.93)
  other vias: 66.04,68.58
N$335  (via drill 0.9 pad 1.93)
  other vias: 66.04,71.12
N$337  (via drill 0.9 pad 1.93)
  other vias: 66.04,73.66
N$338  (via drill 0.9 pad 1.93)
  other vias: 66.04,76.2
N$339  (via drill 0.9 pad 1.93)
  other vias: 63.5,76.2
N$343  (via drill 0.9 pad 1.93)
  other vias: 63.5,73.66
N$344  (via drill 0.9 pad 1.93)
  other vias: 63.5,71.12
N$345  (via drill 0.9 pad 1.93)
  other vias: 63.5,68.58
N$346  (via drill 0.9 pad 1.93)
  other vias: 63.5,66.04
N$349  (via drill 0.9 pad 1.93)
  other vias: 63.5,63.5
N$350  (via drill 0.9 pad 1.93)
  other vias: 40.64,53.34
N$351  (via drill 0.9 pad 1.93)
  other vias: 63.5,58.42
N$352  (via drill 0.9 pad 1.93)
  other vias: 63.5,55.88
N$353  (via drill 0.9 pad 1.93)
  other vias: 60.96,55.88
N$354  (via drill 0.9 pad 1.93)
  other vias: 60.96,58.42
N$356  (via drill 0.9 pad 1.93)
  other vias: 40.64,50.8
N$358  (via drill 0.9 pad 1.93)
  other vias: 60.96,63.5
N$359  (via drill 0.9 pad 1.93)
  other vias: 60.96,66.04
N$361  (via drill 0.9 pad 1.93)
  other vias: 60.96,68.58
N$364  (via drill 0.9 pad 1.93)
  other vias: 60.96,71.12
N$365  (via drill 0.9 pad 1.93)
  other vias: 60.96,73.66
N$366  (via drill 0.9 pad 1.93)
  other vias: 60.96,76.2
N$367  (via drill 0.9 pad 1.93)
  other vias: 58.42,76.2
N$368  (via drill 0.9 pad 1.93)
  other vias: 58.42,73.66
N$369  (via drill 0.9 pad 1.93)
  other vias: 58.42,71.12
N$370  (via drill 0.9 pad 1.93)
  other vias: 58.42,68.58
N$371  (via drill 0.9 pad 1.93)
  other vias: 58.42,66.04
N$372  (via drill 0.9 pad 1.93)
  other vias: 58.42,63.5
N$373  (via drill 0.9 pad 1.93)
  other vias: 40.64,60.96
N$374  (via drill 0.9 pad 1.93)
  other vias: 58.42,58.42
N$375  (via drill 0.9 pad 1.93)
  other vias: 58.42,55.88
N$376  (via drill 0.9 pad 1.93)
  other vias: 55.88,55.88
N$377  (via drill 0.9 pad 1.93)
  other vias: 55.88,58.42
N$378  (via drill 0.9 pad 1.93)
  other vias: 38.1,60.96
N$379  (via drill 0.9 pad 1.93)
  other vias: 55.88,63.5
N$380  (via drill 0.9 pad 1.93)
  other vias: 55.88,66.04
N$381  (via drill 0.9 pad 1.93)
  other vias: 55.88,68.58
N$382  (via drill 0.9 pad 1.93)
  other vias: 55.88,71.12
N$383  (via drill 0.9 pad 1.93)
  other vias: 55.88,73.66
N$384  (via drill 0.9 pad 1.93)
  other vias: 55.88,76.2
N$385  (via drill 0.9 pad 1.93)
  other vias: 53.34,76.2
N$386  (via drill 0.9 pad 1.93)
  other vias: 53.34,73.66
N$387  (via drill 0.9 pad 1.93)
  other vias: 53.34,71.12
N$388  (via drill 0.9 pad 1.93)
  other vias: 53.34,68.58
N$389  (via drill 0.9 pad 1.93)
  other vias: 53.34,66.04
N$390  (via drill 0.9 pad 1.93)
  other vias: 53.34,63.5
N$391  (via drill 0.9 pad 1.93)
  other vias: 35.56,60.96
N$392  (via drill 0.9 pad 1.93)
  other vias: 53.34,58.42
N$393  (via drill 0.9 pad 1.93)
  other vias: 53.34,55.88
N$394  (via drill 0.9 pad 1.93)
  other vias: 50.8,55.88
N$395  (via drill 0.9 pad 1.93)
  other vias: 50.8,58.42
N$396  (via drill 0.9 pad 1.93)
  other vias: 33.02,60.96
N$397  (via drill 0.9 pad 1.93)
  other vias: 50.8,63.5
N$398  (via drill 0.9 pad 1.93)
  other vias: 50.8,66.04
N$399  (via drill 0.9 pad 1.93)
  other vias: 50.8,68.58
N$400  (via drill 0.9 pad 1.93)
  other vias: 50.8,71.12
N$401  (via drill 0.9 pad 1.93)
  other vias: 50.8,73.66
N$402  (via drill 0.9 pad 1.93)
  other vias: 50.8,76.2
N$403  (via drill 0.9 pad 1.93)
  other vias: 48.26,76.2
N$404  (via drill 0.9 pad 1.93)
  other vias: 48.26,73.66
N$405  (via drill 0.9 pad 1.93)
  other vias: 48.26,71.12
N$406  (via drill 0.9 pad 1.93)
  other vias: 48.26,68.58
N$407  (via drill 0.9 pad 1.93)
  other vias: 48.26,66.04
N$408  (via drill 0.9 pad 1.93)
  other vias: 48.26,63.5
N$409  (via drill 0.9 pad 1.93)
  other vias: 30.48,60.96
N$410  (via drill 0.9 pad 1.93)
  other vias: 48.26,58.42
N$411  (via drill 0.9 pad 1.93)
  other vias: 48.26,55.88
N$412  (via drill 0.9 pad 1.93)
  other vias: 27.94,60.96
N$413  (via drill 0.9 pad 1.93)
  other vias: 25.4,60.96
N$414  (via drill 0.9 pad 1.93)
  other vias: 22.86,60.96
N$415  (via drill 0.9 pad 1.93)
  other vias: 20.32,60.96
N$416  (via drill 0.9 pad 1.93)
  other vias: 17.78,60.96
N$417  (via drill 0.9 pad 1.93)
  other vias: 15.24,60.96
N$418  (via drill 0.9 pad 1.93)
  other vias: 12.7,60.96
N$419  (via drill 0.9 pad 1.93)
  other vias: 10.16,60.96
N$420  (via drill 0.9 pad 1.93)
  other vias: 7.62,60.96
N$421  (via drill 0.9 pad 1.93)
  other vias: 5.08,60.96
N$422  (via drill 0.9 pad 1.93)
  other vias: 40.64,27.94
N$423  (via drill 0.9 pad 1.93)
  other vias: 38.1,27.94
N$424  (via drill 0.9 pad 1.93)
  other vias: 35.56,27.94
N$425  (via drill 0.9 pad 1.93)
  other vias: 33.02,27.94
N$426  (via drill 0.9 pad 1.93)
  other vias: 30.48,27.94
N$427  (via drill 0.9 pad 1.93)
  other vias: 27.94,27.94
N$428  (via drill 0.9 pad 1.93)
  other vias: 25.4,27.94
N$429  (via drill 0.9 pad 1.93)
  other vias: 22.86,27.94
N$430  (via drill 0.9 pad 1.93)
  other vias: 40.64,55.88
N$431  (via drill 0.9 pad 1.93)
  other vias: 20.32,27.94
N$432  (via drill 0.9 pad 1.93)
  other vias: 17.78,27.94
N$433  (via drill 0.9 pad 1.93)
  other vias: 40.64,63.5
N$434  (via drill 0.9 pad 1.93)
  other vias: 40.64,66.04
N$435  (via drill 0.9 pad 1.93)
  other vias: 40.64,68.58
N$436  (via drill 0.9 pad 1.93)
  other vias: 40.64,71.12
N$437  (via drill 0.9 pad 1.93)
  other vias: 40.64,73.66
N$438  (via drill 0.9 pad 1.93)
  other vias: 40.64,76.2
N$439  (via drill 0.9 pad 1.93)
  other vias: 38.1,76.2
N$440  (via drill 0.9 pad 1.93)
  other vias: 38.1,73.66
N$441  (via drill 0.9 pad 1.93)
  other vias: 38.1,71.12
N$442  (via drill 0.9 pad 1.93)
  other vias: 38.1,68.58
N$443  (via drill 0.9 pad 1.93)
  other vias: 38.1,66.04
N$444  (via drill 0.9 pad 1.93)
  other vias: 38.1,63.5
N$445  (via drill 0.9 pad 1.93)
  other vias: 15.24,27.94
N$446  (via drill 0.9 pad 1.93)
  other vias: 38.1,58.42
N$447  (via drill 0.9 pad 1.93)
  other vias: 38.1,55.88
N$448  (via drill 0.9 pad 1.93)
  other vias: 35.56,55.88
N$449  (via drill 0.9 pad 1.93)
  other vias: 35.56,58.42
N$450  (via drill 0.9 pad 1.93)
  other vias: 12.7,27.94
N$451  (via drill 0.9 pad 1.93)
  other vias: 35.56,63.5
N$452  (via drill 0.9 pad 1.93)
  other vias: 35.56,66.04
N$453  (via drill 0.9 pad 1.93)
  other vias: 35.56,68.58
N$454  (via drill 0.9 pad 1.93)
  other vias: 35.56,71.12
N$455  (via drill 0.9 pad 1.93)
  other vias: 35.56,73.66
N$456  (via drill 0.9 pad 1.93)
  other vias: 35.56,76.2
N$457  (via drill 0.9 pad 1.93)
  other vias: 33.02,76.2
N$458  (via drill 0.9 pad 1.93)
  other vias: 33.02,73.66
N$459  (via drill 0.9 pad 1.93)
  other vias: 33.02,71.12
N$460  (via drill 0.9 pad 1.93)
  other vias: 33.02,68.58
N$461  (via drill 0.9 pad 1.93)
  other vias: 33.02,66.04
N$462  (via drill 0.9 pad 1.93)
  other vias: 33.02,63.5
N$463  (via drill 0.9 pad 1.93)
  other vias: 10.16,27.94
N$464  (via drill 0.9 pad 1.93)
  other vias: 33.02,58.42
N$465  (via drill 0.9 pad 1.93)
  other vias: 33.02,55.88
N$466  (via drill 0.9 pad 1.93)
  other vias: 30.48,55.88
N$467  (via drill 0.9 pad 1.93)
  other vias: 30.48,58.42
N$468  (via drill 0.9 pad 1.93)
  other vias: 7.62,27.94
N$469  (via drill 0.9 pad 1.93)
  other vias: 30.48,63.5
N$470  (via drill 0.9 pad 1.93)
  other vias: 30.48,66.04
N$471  (via drill 0.9 pad 1.93)
  other vias: 30.48,68.58
N$472  (via drill 0.9 pad 1.93)
  other vias: 30.48,71.12
N$473  (via drill 0.9 pad 1.93)
  other vias: 30.48,73.66
N$474  (via drill 0.9 pad 1.93)
  other vias: 30.48,76.2
N$475  (via drill 0.9 pad 1.93)
  other vias: 27.94,76.2
N$476  (via drill 0.9 pad 1.93)
  other vias: 27.94,73.66
N$477  (via drill 0.9 pad 1.93)
  other vias: 27.94,71.12
N$478  (via drill 0.9 pad 1.93)
  other vias: 27.94,68.58
N$479  (via drill 0.9 pad 1.93)
  other vias: 27.94,66.04
N$480  (via drill 0.9 pad 1.93)
  other vias: 27.94,63.5
N$481  (via drill 0.9 pad 1.93)
  other vias: 5.08,27.94
N$482  (via drill 0.9 pad 1.93)
  other vias: 27.94,58.42
N$483  (via drill 0.9 pad 1.93)
  other vias: 27.94,55.88
N$484  (via drill 0.9 pad 1.93)
  other vias: 25.4,55.88
N$485  (via drill 0.9 pad 1.93)
  other vias: 25.4,58.42
N$486  (via drill 0.9 pad 1.93)
  other vias: 40.64,81.28
N$487  (via drill 0.9 pad 1.93)
  other vias: 25.4,63.5
N$488  (via drill 0.9 pad 1.93)
  other vias: 25.4,66.04
N$489  (via drill 0.9 pad 1.93)
  other vias: 25.4,68.58
N$490  (via drill 0.9 pad 1.93)
  other vias: 25.4,71.12
N$491  (via drill 0.9 pad 1.93)
  other vias: 25.4,73.66
N$492  (via drill 0.9 pad 1.93)
  other vias: 25.4,76.2
N$493  (via drill 0.9 pad 1.93)
  other vias: 22.86,76.2
N$494  (via drill 0.9 pad 1.93)
  other vias: 22.86,73.66
N$495  (via drill 0.9 pad 1.93)
  other vias: 22.86,71.12
N$496  (via drill 0.9 pad 1.93)
  other vias: 22.86,68.58
N$497  (via drill 0.9 pad 1.93)
  other vias: 22.86,66.04
N$498  (via drill 0.9 pad 1.93)
  other vias: 22.86,63.5
N$499  (via drill 0.9 pad 1.93)
  other vias: 40.64,83.82
N$500  (via drill 0.9 pad 1.93)
  other vias: 22.86,58.42
N$501  (via drill 0.9 pad 1.93)
  other vias: 22.86,55.88
N$502  (via drill 0.9 pad 1.93)
  other vias: 20.32,55.88
N$503  (via drill 0.9 pad 1.93)
  other vias: 20.32,58.42
N$504  (via drill 0.9 pad 1.93)
  other vias: 40.64,86.36
N$505  (via drill 0.9 pad 1.93)
  other vias: 20.32,63.5
N$506  (via drill 0.9 pad 1.93)
  other vias: 20.32,66.04
N$507  (via drill 0.9 pad 1.93)
  other vias: 20.32,68.58
N$508  (via drill 0.9 pad 1.93)
  other vias: 20.32,71.12
N$509  (via drill 0.9 pad 1.93)
  other vias: 20.32,73.66
N$510  (via drill 0.9 pad 1.93)
  other vias: 20.32,76.2
N$511  (via drill 0.9 pad 1.93)
  other vias: 17.78,76.2
N$512  (via drill 0.9 pad 1.93)
  other vias: 17.78,73.66
N$513  (via drill 0.9 pad 1.93)
  other vias: 17.78,71.12
N$514  (via drill 0.9 pad 1.93)
  other vias: 17.78,68.58
N$515  (via drill 0.9 pad 1.93)
  other vias: 17.78,66.04
N$516  (via drill 0.9 pad 1.93)
  other vias: 17.78,63.5
N$517  (via drill 0.9 pad 1.93)
  other vias: 40.64,88.9
N$518  (via drill 0.9 pad 1.93)
  other vias: 17.78,58.42
N$519  (via drill 0.9 pad 1.93)
  other vias: 17.78,55.88
N$520  (via drill 0.9 pad 1.93)
  other vias: 15.24,55.88
N$521  (via drill 0.9 pad 1.93)
  other vias: 15.24,58.42
N$522  (via drill 0.9 pad 1.93)
  other vias: 40.64,91.44
N$523  (via drill 0.9 pad 1.93)
  other vias: 15.24,63.5
N$524  (via drill 0.9 pad 1.93)
  other vias: 15.24,66.04
N$525  (via drill 0.9 pad 1.93)
  other vias: 15.24,68.58
N$526  (via drill 0.9 pad 1.93)
  other vias: 15.24,71.12
N$527  (via drill 0.9 pad 1.93)
  other vias: 15.24,73.66
N$528  (via drill 0.9 pad 1.93)
  other vias: 15.24,76.2
N$529  (via drill 0.9 pad 1.93)
  other vias: 12.7,76.2
N$530  (via drill 0.9 pad 1.93)
  other vias: 12.7,73.66
N$531  (via drill 0.9 pad 1.93)
  other vias: 12.7,71.12
N$532  (via drill 0.9 pad 1.93)
  other vias: 12.7,68.58
N$533  (via drill 0.9 pad 1.93)
  other vias: 12.7,66.04
N$534  (via drill 0.9 pad 1.93)
  other vias: 12.7,63.5
N$535  (via drill 0.9 pad 1.93)
  other vias: 38.1,91.44
N$536  (via drill 0.9 pad 1.93)
  other vias: 12.7,58.42
N$537  (via drill 0.9 pad 1.93)
  other vias: 12.7,55.88
N$538  (via drill 0.9 pad 1.93)
  other vias: 10.16,55.88
N$539  (via drill 0.9 pad 1.93)
  other vias: 10.16,58.42
N$540  (via drill 0.9 pad 1.93)
  other vias: 38.1,88.9
N$541  (via drill 0.9 pad 1.93)
  other vias: 10.16,63.5
N$542  (via drill 0.9 pad 1.93)
  other vias: 10.16,66.04
N$543  (via drill 0.9 pad 1.93)
  other vias: 10.16,68.58
N$544  (via drill 0.9 pad 1.93)
  other vias: 10.16,71.12
N$545  (via drill 0.9 pad 1.93)
  other vias: 10.16,73.66
N$546  (via drill 0.9 pad 1.93)
  other vias: 10.16,76.2
N$547  (via drill 0.9 pad 1.93)
  other vias: 38.1,86.36
N$548  (via drill 0.9 pad 1.93)
  other vias: 86.36,76.2
N$549  (via drill 0.9 pad 1.93)
  other vias: 86.36,73.66
N$551  (via drill 0.9 pad 1.93)
  other vias: 86.36,71.12
N$553  (via drill 0.9 pad 1.93)
  other vias: 27.94,48.26
N$554  (via drill 0.9 pad 1.93)
  other vias: 27.94,45.72
N$555  (via drill 0.9 pad 1.93)
  other vias: 27.94,43.18
N$556  (via drill 0.9 pad 1.93)
  other vias: 27.94,40.64
N$557  (via drill 0.9 pad 1.93)
  other vias: 27.94,38.1
N$558  (via drill 0.9 pad 1.93)
  other vias: 27.94,35.56
N$559  (via drill 0.9 pad 1.93)
  other vias: 27.94,33.02
N$560  (via drill 0.9 pad 1.93)
  other vias: 27.94,30.48
N$561  (via drill 0.9 pad 1.93)
  other vias: 38.1,83.82
N$562  (via drill 0.9 pad 1.93)
  other vias: 38.1,81.28
N$563  (via drill 0.9 pad 1.93)
  other vias: 25.4,30.48
N$564  (via drill 0.9 pad 1.93)
  other vias: 25.4,33.02
N$565  (via drill 0.9 pad 1.93)
  other vias: 25.4,35.56
N$566  (via drill 0.9 pad 1.93)
  other vias: 25.4,38.1
N$567  (via drill 0.9 pad 1.93)
  other vias: 25.4,40.64
N$568  (via drill 0.9 pad 1.93)
  other vias: 25.4,43.18
N$569  (via drill 0.9 pad 1.93)
  other vias: 25.4,45.72
N$570  (via drill 0.9 pad 1.93)
  other vias: 25.4,48.26
N$571  (via drill 0.9 pad 1.93)
  other vias: 22.86,48.26
N$572  (via drill 0.9 pad 1.93)
  other vias: 22.86,45.72
N$573  (via drill 0.9 pad 1.93)
  other vias: 22.86,43.18
N$574  (via drill 0.9 pad 1.93)
  other vias: 22.86,40.64
N$575  (via drill 0.9 pad 1.93)
  other vias: 22.86,38.1
N$576  (via drill 0.9 pad 1.93)
  other vias: 22.86,35.56
N$577  (via drill 0.9 pad 1.93)
  other vias: 22.86,33.02
N$578  (via drill 0.9 pad 1.93)
  other vias: 22.86,30.48
N$579  (via drill 0.9 pad 1.93)
  other vias: 38.1,78.74
N$580  (via drill 0.9 pad 1.93)
  other vias: 35.56,78.74
N$581  (via drill 0.9 pad 1.93)
  other vias: 20.32,30.48
N$582  (via drill 0.9 pad 1.93)
  other vias: 20.32,33.02
N$583  (via drill 0.9 pad 1.93)
  other vias: 20.32,35.56
N$584  (via drill 0.9 pad 1.93)
  other vias: 20.32,38.1
N$585  (via drill 0.9 pad 1.93)
  other vias: 20.32,40.64
N$586  (via drill 0.9 pad 1.93)
  other vias: 20.32,43.18
N$587  (via drill 0.9 pad 1.93)
  other vias: 20.32,45.72
N$588  (via drill 0.9 pad 1.93)
  other vias: 20.32,48.26
N$589  (via drill 0.9 pad 1.93)
  other vias: 17.78,48.26
N$590  (via drill 0.9 pad 1.93)
  other vias: 17.78,45.72
N$591  (via drill 0.9 pad 1.93)
  other vias: 17.78,43.18
N$592  (via drill 0.9 pad 1.93)
  other vias: 17.78,40.64
N$593  (via drill 0.9 pad 1.93)
  other vias: 17.78,38.1
N$594  (via drill 0.9 pad 1.93)
  other vias: 17.78,35.56
N$595  (via drill 0.9 pad 1.93)
  other vias: 17.78,33.02
N$596  (via drill 0.9 pad 1.93)
  other vias: 17.78,30.48
N$597  (via drill 0.9 pad 1.93)
  other vias: 35.56,81.28
N$598  (via drill 0.9 pad 1.93)
  other vias: 35.56,83.82
N$599  (via drill 0.9 pad 1.93)
  other vias: 15.24,30.48
N$600  (via drill 0.9 pad 1.93)
  other vias: 15.24,33.02
N$601  (via drill 0.9 pad 1.93)
  other vias: 15.24,35.56
N$602  (via drill 0.9 pad 1.93)
  other vias: 15.24,38.1
N$603  (via drill 0.9 pad 1.93)
  other vias: 15.24,40.64
N$604  (via drill 0.9 pad 1.93)
  other vias: 15.24,43.18
N$605  (via drill 0.9 pad 1.93)
  other vias: 15.24,45.72
N$606  (via drill 0.9 pad 1.93)
  other vias: 15.24,48.26
N$607  (via drill 0.9 pad 1.93)
  other vias: 27.94,25.4
N$608  (via drill 0.9 pad 1.93)
  other vias: 27.94,22.86
N$609  (via drill 0.9 pad 1.93)
  other vias: 27.94,20.32
N$610  (via drill 0.9 pad 1.93)
  other vias: 27.94,17.78
N$611  (via drill 0.9 pad 1.93)
  other vias: 27.94,15.24
N$612  (via drill 0.9 pad 1.93)
  other vias: 27.94,12.7
N$613  (via drill 0.9 pad 1.93)
  other vias: 27.94,10.16
N$614  (via drill 0.9 pad 1.93)
  other vias: 27.94,7.62
N$615  (via drill 0.9 pad 1.93)
  other vias: 27.94,5.08
N$616  (via drill 0.9 pad 1.93)
  other vias: 25.4,5.08
N$617  (via drill 0.9 pad 1.93)
  other vias: 25.4,7.62
N$618  (via drill 0.9 pad 1.93)
  other vias: 25.4,10.16
N$619  (via drill 0.9 pad 1.93)
  other vias: 25.4,12.7
N$620  (via drill 0.9 pad 1.93)
  other vias: 25.4,15.24
N$621  (via drill 0.9 pad 1.93)
  other vias: 25.4,17.78
N$622  (via drill 0.9 pad 1.93)
  other vias: 25.4,20.32
N$623  (via drill 0.9 pad 1.93)
  other vias: 25.4,22.86
N$624  (via drill 0.9 pad 1.93)
  other vias: 25.4,25.4
N$625  (via drill 0.9 pad 1.93)
  other vias: 22.86,25.4
N$626  (via drill 0.9 pad 1.93)
  other vias: 22.86,22.86
N$627  (via drill 0.9 pad 1.93)
  other vias: 22.86,20.32
N$628  (via drill 0.9 pad 1.93)
  other vias: 22.86,17.78
N$629  (via drill 0.9 pad 1.93)
  other vias: 22.86,15.24
N$630  (via drill 0.9 pad 1.93)
  other vias: 22.86,12.7
N$631  (via drill 0.9 pad 1.93)
  other vias: 22.86,10.16
N$632  (via drill 0.9 pad 1.93)
  other vias: 22.86,7.62
N$633  (via drill 0.9 pad 1.93)
  other vias: 22.86,5.08
N$634  (via drill 0.9 pad 1.93)
  other vias: 20.32,5.08
N$635  (via drill 0.9 pad 1.93)
  other vias: 20.32,7.62
N$636  (via drill 0.9 pad 1.93)
  other vias: 20.32,10.16
N$637  (via drill 0.9 pad 1.93)
  other vias: 20.32,12.7
N$638  (via drill 0.9 pad 1.93)
  other vias: 20.32,15.24
N$639  (via drill 0.9 pad 1.93)
  other vias: 20.32,17.78
N$640  (via drill 0.9 pad 1.93)
  other vias: 20.32,20.32
N$641  (via drill 0.9 pad 1.93)
  other vias: 20.32,22.86
N$642  (via drill 0.9 pad 1.93)
  other vias: 20.32,25.4
N$643  (via drill 0.9 pad 1.93)
  other vias: 17.78,25.4
N$644  (via drill 0.9 pad 1.93)
  other vias: 17.78,22.86
N$645  (via drill 0.9 pad 1.93)
  other vias: 17.78,20.32
N$646  (via drill 0.9 pad 1.93)
  other vias: 17.78,17.78
N$647  (via drill 0.9 pad 1.93)
  other vias: 17.78,15.24
N$648  (via drill 0.9 pad 1.93)
  other vias: 17.78,12.7
N$649  (via drill 0.9 pad 1.93)
  other vias: 17.78,10.16
N$650  (via drill 0.9 pad 1.93)
  other vias: 17.78,7.62
N$651  (via drill 0.9 pad 1.93)
  other vias: 17.78,5.08
N$652  (via drill 0.9 pad 1.93)
  other vias: 15.24,5.08
N$653  (via drill 0.9 pad 1.93)
  other vias: 15.24,7.62
N$654  (via drill 0.9 pad 1.93)
  other vias: 15.24,10.16
N$655  (via drill 0.9 pad 1.93)
  other vias: 15.24,12.7
N$656  (via drill 0.9 pad 1.93)
  other vias: 15.24,15.24
N$657  (via drill 0.9 pad 1.93)
  other vias: 15.24,17.78
N$658  (via drill 0.9 pad 1.93)
  other vias: 15.24,20.32
N$661  (via drill 0.9 pad 1.93)
  other vias: 15.24,22.86
N$662  (via drill 0.9 pad 1.93)
  other vias: 15.24,25.4
N$663  (via drill 0.9 pad 1.93)
  other vias: 86.36,68.58
N$665  (via drill 0.9 pad 1.93)
  other vias: 86.36,66.04
N$666  (via drill 0.9 pad 1.93)
  other vias: 86.36,63.5
N$667  (via drill 0.9 pad 1.93)
  other vias: 86.36,58.42
N$668  (via drill 0.9 pad 1.93)
  other vias: 86.36,55.88
N$669  (via drill 0.9 pad 1.93)
  other vias: 7.62,55.88
N$670  (via drill 0.9 pad 1.93)
  other vias: 7.62,58.42
N$671  (via drill 0.9 pad 1.93)
  other vias: 35.56,86.36
N$672  (via drill 0.9 pad 1.93)
  other vias: 7.62,63.5
N$673  (via drill 0.9 pad 1.93)
  other vias: 7.62,66.04
N$674  (via drill 0.9 pad 1.93)
  other vias: 7.62,68.58
N$675  (via drill 0.9 pad 1.93)
  other vias: 7.62,71.12
N$676  (via drill 0.9 pad 1.93)
  other vias: 7.62,73.66
N$677  (via drill 0.9 pad 1.93)
  other vias: 7.62,76.2
N$678  (via drill 0.9 pad 1.93)
  other vias: 5.08,55.88
N$679  (via drill 0.9 pad 1.93)
  other vias: 5.08,58.42
N$680  (via drill 0.9 pad 1.93)
  other vias: 35.56,88.9
N$681  (via drill 0.9 pad 1.93)
  other vias: 5.08,63.5
N$682  (via drill 0.9 pad 1.93)
  other vias: 5.08,66.04
N$683  (via drill 0.9 pad 1.93)
  other vias: 5.08,68.58
N$684  (via drill 0.9 pad 1.93)
  other vias: 5.08,71.12
N$685  (via drill 0.9 pad 1.93)
  other vias: 12.7,48.26
N$686  (via drill 0.9 pad 1.93)
  other vias: 12.7,45.72
N$687  (via drill 0.9 pad 1.93)
  other vias: 12.7,43.18
N$688  (via drill 0.9 pad 1.93)
  other vias: 12.7,40.64
N$689  (via drill 0.9 pad 1.93)
  other vias: 12.7,38.1
N$690  (via drill 0.9 pad 1.93)
  other vias: 12.7,35.56
N$691  (via drill 0.9 pad 1.93)
  other vias: 12.7,33.02
N$692  (via drill 0.9 pad 1.93)
  other vias: 12.7,30.48
N$693  (via drill 0.9 pad 1.93)
  other vias: 35.56,91.44
N$694  (via drill 0.9 pad 1.93)
  other vias: 33.02,91.44
N$695  (via drill 0.9 pad 1.93)
  other vias: 10.16,30.48
N$696  (via drill 0.9 pad 1.93)
  other vias: 10.16,33.02
N$697  (via drill 0.9 pad 1.93)
  other vias: 10.16,35.56
N$698  (via drill 0.9 pad 1.93)
  other vias: 10.16,38.1
N$699  (via drill 0.9 pad 1.93)
  other vias: 10.16,40.64
N$700  (via drill 0.9 pad 1.93)
  other vias: 10.16,43.18
N$701  (via drill 0.9 pad 1.93)
  other vias: 10.16,45.72
N$702  (via drill 0.9 pad 1.93)
  other vias: 10.16,48.26
N$703  (via drill 0.9 pad 1.93)
  other vias: 7.62,48.26
N$704  (via drill 0.9 pad 1.93)
  other vias: 7.62,45.72
N$705  (via drill 0.9 pad 1.93)
  other vias: 7.62,43.18
N$706  (via drill 0.9 pad 1.93)
  other vias: 7.62,40.64
N$707  (via drill 0.9 pad 1.93)
  other vias: 7.62,38.1
N$708  (via drill 0.9 pad 1.93)
  other vias: 7.62,35.56
N$709  (via drill 0.9 pad 1.93)
  other vias: 7.62,33.02
N$710  (via drill 0.9 pad 1.93)
  other vias: 7.62,30.48
N$711  (via drill 0.9 pad 1.93)
  other vias: 33.02,88.9
N$712  (via drill 0.9 pad 1.93)
  other vias: 33.02,86.36
N$713  (via drill 0.9 pad 1.93)
  other vias: 5.08,30.48
N$714  (via drill 0.9 pad 1.93)
  other vias: 5.08,33.02
N$715  (via drill 0.9 pad 1.93)
  other vias: 5.08,35.56
N$716  (via drill 0.9 pad 1.93)
  other vias: 5.08,38.1
N$717  (via drill 0.9 pad 1.93)
  other vias: 5.08,40.64
N$718  (via drill 0.9 pad 1.93)
  other vias: 5.08,43.18
N$719  (via drill 0.9 pad 1.93)
  other vias: 5.08,45.72
N$720  (via drill 0.9 pad 1.93)
  other vias: 5.08,48.26
N$721  (via drill 0.9 pad 1.93)
  other vias: 12.7,25.4
N$722  (via drill 0.9 pad 1.93)
  other vias: 12.7,22.86
N$723  (via drill 0.9 pad 1.93)
  other vias: 12.7,20.32
N$724  (via drill 0.9 pad 1.93)
  other vias: 12.7,17.78
N$725  (via drill 0.9 pad 1.93)
  other vias: 12.7,15.24
N$726  (via drill 0.9 pad 1.93)
  other vias: 12.7,12.7
N$727  (via drill 0.9 pad 1.93)
  other vias: 12.7,10.16
N$728  (via drill 0.9 pad 1.93)
  other vias: 12.7,7.62
N$729  (via drill 0.9 pad 1.93)
  other vias: 12.7,5.08
N$730  (via drill 0.9 pad 1.93)
  other vias: 10.16,5.08
N$731  (via drill 0.9 pad 1.93)
  other vias: 10.16,7.62
N$732  (via drill 0.9 pad 1.93)
  other vias: 10.16,10.16
N$733  (via drill 0.9 pad 1.93)
  other vias: 10.16,12.7
N$734  (via drill 0.9 pad 1.93)
  other vias: 10.16,15.24
N$735  (via drill 0.9 pad 1.93)
  other vias: 10.16,17.78
N$736  (via drill 0.9 pad 1.93)
  other vias: 10.16,20.32
N$737  (via drill 0.9 pad 1.93)
  other vias: 10.16,22.86
N$738  (via drill 0.9 pad 1.93)
  other vias: 10.16,25.4
N$739  (via drill 0.9 pad 1.93)
  other vias: 7.62,25.4
N$740  (via drill 0.9 pad 1.93)
  other vias: 7.62,22.86
N$741  (via drill 0.9 pad 1.93)
  other vias: 7.62,20.32
N$742  (via drill 0.9 pad 1.93)
  other vias: 7.62,17.78
N$743  (via drill 0.9 pad 1.93)
  other vias: 7.62,15.24
N$744  (via drill 0.9 pad 1.93)
  other vias: 7.62,12.7
N$745  (via drill 0.9 pad 1.93)
  other vias: 7.62,10.16
N$746  (via drill 0.9 pad 1.93)
  other vias: 7.62,7.62
N$747  (via drill 0.9 pad 1.93)
  other vias: 7.62,5.08
N$748  (via drill 0.9 pad 1.93)
  other vias: 33.02,83.82
N$749  (via drill 0.9 pad 1.93)
  other vias: 33.02,81.28
N$750  (via drill 0.9 pad 1.93)
  other vias: 5.08,10.16
N$751  (via drill 0.9 pad 1.93)
  other vias: 5.08,12.7
N$752  (via drill 0.9 pad 1.93)
  other vias: 5.08,15.24
N$753  (via drill 0.9 pad 1.93)
  other vias: 5.08,17.78
N$754  (via drill 0.9 pad 1.93)
  other vias: 5.08,20.32
N$755  (via drill 0.9 pad 1.93)
  other vias: 5.08,22.86
N$756  (via drill 0.9 pad 1.93)
  other vias: 5.08,25.4
N$757  (via drill 0.9 pad 1.93)
  other vias: 86.36,91.44
N$759  (via drill 0.9 pad 1.93)
  other vias: 86.36,88.9
N$760  (via drill 0.9 pad 1.93)
  other vias: 33.02,78.74
N$761  (via drill 0.9 pad 1.93)
  other vias: 30.48,78.74
N$762  (via drill 0.9 pad 1.93)
  other vias: 30.48,81.28
N$763  (via drill 0.9 pad 1.93)
  other vias: 30.48,83.82
N$764  (via drill 0.9 pad 1.93)
  other vias: 30.48,86.36
N$765  (via drill 0.9 pad 1.93)
  other vias: 30.48,88.9
N$766  (via drill 0.9 pad 1.93)
  other vias: 30.48,91.44
N$767  (via drill 0.9 pad 1.93)
  other vias: 27.94,91.44
N$768  (via drill 0.9 pad 1.93)
  other vias: 27.94,88.9
N$769  (via drill 0.9 pad 1.93)
  other vias: 27.94,86.36
N$770  (via drill 0.9 pad 1.93)
  other vias: 27.94,83.82
N$771  (via drill 0.9 pad 1.93)
  other vias: 27.94,81.28
N$772  (via drill 0.9 pad 1.93)
  other vias: 27.94,78.74
N$773  (via drill 0.9 pad 1.93)
  other vias: 25.4,78.74
N$774  (via drill 0.9 pad 1.93)
  other vias: 25.4,81.28
N$775  (via drill 0.9 pad 1.93)
  other vias: 25.4,83.82
N$776  (via drill 0.9 pad 1.93)
  other vias: 25.4,86.36
N$777  (via drill 0.9 pad 1.93)
  other vias: 25.4,88.9
N$778  (via drill 0.9 pad 1.93)
  other vias: 25.4,91.44
N$779  (via drill 0.9 pad 1.93)
  other vias: 22.86,91.44
N$780  (via drill 0.9 pad 1.93)
  other vias: 22.86,88.9
N$781  (via drill 0.9 pad 1.93)
  other vias: 22.86,86.36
